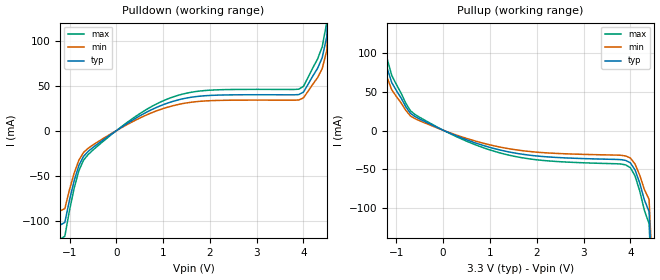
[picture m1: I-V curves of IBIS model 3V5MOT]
[IBIS Ver]   2.1
[File name]   171401_3.ibs
[File Rev]   2.0
[Date]   03/17/1999
[Source]   ICS MicroClock Applications Engineering 2
[Disclaimer] This information is for modeling purposes only, and is
(C) Copyright Integrated Circuit Systems, Inc. 1997-2001
   All rights reserved
ICS hereby grants the user of this IBIS model a non-exclusive,
nontransferable license to use this IBIS model under the following terms.
Before using this IBIS model, the user should read this license.
If the user does not accept these terms,  the IBIS model should be
returned to ICS within 30 days.
   The user is granted this license only to use the IBIS model and
is not granted rights to sell, load, rent, lease or license the IBIS
model in whole or in part, or in modified form to anyone other than
user. User may modify the IBIS model to suit its specific
applications but rights to derivative works and such modifications
shall belong to ICS.
   This IBIS model is provided on an "AS IS" basis and ICS makes
absolutely no warranty with respect to the information contained
herein. ICS DISCLAIMS AND CUSTOMER WAIVES ALL WARRANTIES, EXPRESS
OR IMPLIED, INCLUDING WARRANTIES OF MERCHANTABILITY OR FITNESS FOR
A PARTICULAR PURPOSE. The entire risk as to quality and performance
is with the Customer. ACCORDINGLY, IN NO EVENT SHALL THE COMPANY BE
LIABLE FOR ANY DAMAGES, WHETHER IN CONTRACT OR TORT,INCLUDING ANY
LOST PROFITS OR OTHER INCIDENTAL, CONSEQUENTIAL, EXEMPLARY, OR
PUNITIVE DAMAGES ARISING OUT OF THE USE OR APPLICATION OF THE IBIS
model provided in this package. Further, ICS reserves the right to
make changes without notice to any product herein to improve
reliability, function, or design. ICS does not convey any license
under patent rights or any other intellectual property rights,
including those of third parties.
   ICS is not obligated to provide maintenance or support
for the licensed IBIS model.
[Component]   MK1714-01
[Manufacturer] Integrated Circuit Systems Inc.
[Package]
|   typ   min   max
R_pkg   40m   35m   45m
L_pkg   1.65nH   1.35nH   1.95nH
C_pkg   0.24pF   0.14pF   0.34pF
[pin]   signal_name   model_name   R_pin   L_pin   C_pin
   20   REF   3V5MOT
   10   CLK   3V5MOT
| Models and submodels in the file (1): 3V5MOT (Output)
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|   MK1714 3.3V Clock Drive Model
| This model is suitable for all single output pins on the
| MK1714 family
[Model]   3V5MOT
Model_type   Output
Polarity   Non-Inverting
|   typ   min   max
C_comp   5pF   4pF   6pF
|   typ   min   max
[Voltage range]  3.3V   3.15V   3.45V
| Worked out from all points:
|   slope of the pulldown table from 0 to 0.495 V, typ, clamps not added: 30.4 ohm
|   slope of the pullup table from 0 to 0.495 V, typ, clamps not added: 40.2 ohm
[pulldown]
|Voltage I (typ)   I (min)   I (max)
-3.3V     -3A        -3A        -3A
-1.1V     -102.1mA   -86.77mA   -117.4mA
-900mV    -55.57mA   -47.23mA   -63.9mA
-700mV    -28.65mA   -24.35mA   -32.95mA
700mV     21.79mA    18.53mA    25.06mA
1.7V      37.66mA    32.02mA    43.31mA
3.9V      39.95mA    33.96mA    45.95mA
4V        42.71mA    36.3mA     49.12mA
4.3V      68.96mA    58.61mA    79.3mA
4.4V      80.83mA    68.71mA    92.96mA
4.5V      105mA      89.25mA    120.7mA
6.6V      3A         3A         3A
[pullup]
|Voltage I (typ)   I (min)   I (max)
-3.3V     3A         3A         3A
-1.3V     105mA      89.25mA    120.7mA
-1.1V     62.23mA    52.9mA     71.57mA
-700mV    22.28mA    18.94mA    25.62mA
-100mV    3.139mA    2.668mA    3.61mA
700mV     -16.3mA    -13.86mA   -18.75mA
1.5V      -28.85mA   -24.52mA   -33.18mA
3.9V      -38.77mA   -32.96mA   -44.59mA
4V        -41.85mA   -35.57mA   -48.13mA
4.1V      -51.12mA   -43.45mA   -58.79mA
4.4V      -105mA     -89.25mA   -120.7mA
6.6V      -3A        -3A        -3A
[Ramp]
|   typ   min   max
dV/dt_r   1.00/1.64n   0.95/1.80n   1.04/1.48n
dV/dt_f   1.16/1.17n   1.10/1.28n   1.22/1.05n
